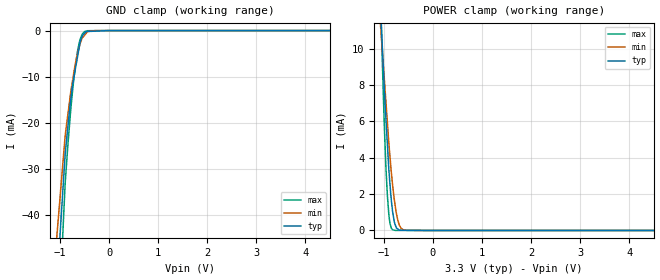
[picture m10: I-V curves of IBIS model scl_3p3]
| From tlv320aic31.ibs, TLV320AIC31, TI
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|   scl_3p3 Model
[Model]   scl_3p3
Model_type   Input
Vinl = 0.99
Vinh = 2.31
|   typ   min   max
|   (nom PVT)   (fast PVT)   (slow PVT)
|C_comp from frequency sweep method (F=400KHz)
|Average
|Average
|C_comp   2.273e-11   2.209e-11   2.278e-11
|C_comp from LC tank measurement(L=1nH)
|Average
|Resonant Frequency(Hz)   2.110e+09   2.120e+09   2.090e+09
C_comp   5.695e-12   5.642e-12   5.805e-12
| Where nom  PVT is Nominal Process, 3.3V, 26C
|   Fast PVT is Strong Process,  3.6V, -40C
|   Slow PVT is Weak Process,   3V, 86C
[Model Spec]
|Subparameter   typ   min   max
Vinl   0.99   0.9   1.08
Vinh   2.31   2.1   2.52
[Voltage Range]   3.3   3   3.6
|Ambient Temperature   25   85   -40
|Junction Temperature
[Temperature Range]   26   86   -40
[Power Clamp Reference]   3.3   3   3.6
[GND Clamp Reference]   0   0   0
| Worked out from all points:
|   GND clamp passes 1 mA (typ) near -0.54 V on its own axis
|   POWER clamp passes 1 mA (typ) near -0.82 V on its own axis
[GND Clamp]
|   Voltage   I(typ)   I(min)   I(max)
-3.3V     -1.344A    -1.13A     -1.633A
-1.447V   -119.4mA   -93.71mA   -159mA
-897.6mV  -26.97mA   -22.95mA   -33.38mA
-842.4mV  -20.97mA   -18.29mA   -25mA
-792mV    -15.83mA   -14.07mA   -18.33mA
-745.8mV  -11.76mA   -10.85mA   -13.05mA
-691.2mV  -8.484mA   -7.38mA    -7.845mA
-601.2mV  -3.078mA   -3.2mA     -2.248mA
-554.4mV  -1.366mA   -1.715mA   -856.1uA
-500.4mV  -566.1uA   -990.5uA   -208.2uA
-285mV    -122.8uA   -4.282uA   -15.3uA
6.6V      0A         0A         0A
[POWER Clamp]
|   Voltage   I(typ)   I(min)   I(max)
-3.3V     157.9mA    110.4mA    274.6mA
-1.089V   13.36mA    12.1mA     15.18mA
-1.037V   10.41mA    10.1mA     9.822mA
-993.6mV  7.977mA    8.451mA    6.026mA
-961.2mV  6.3mA      7.213mA    3.694mA
-928.8mV  4.786mA    5.974mA    1.956mA
-874.8mV  2.533mA    4.048mA    387.6uA
-820.8mV  1.031mA    2.477mA    39.19uA
-785.4mV  455.6uA    1.675mA    15.66uA
-717mV    84.01uA    584.6uA    1.359uA
-591mV    14.18uA    23.34uA    10.03nA
6.6V      0A         0A         0A
